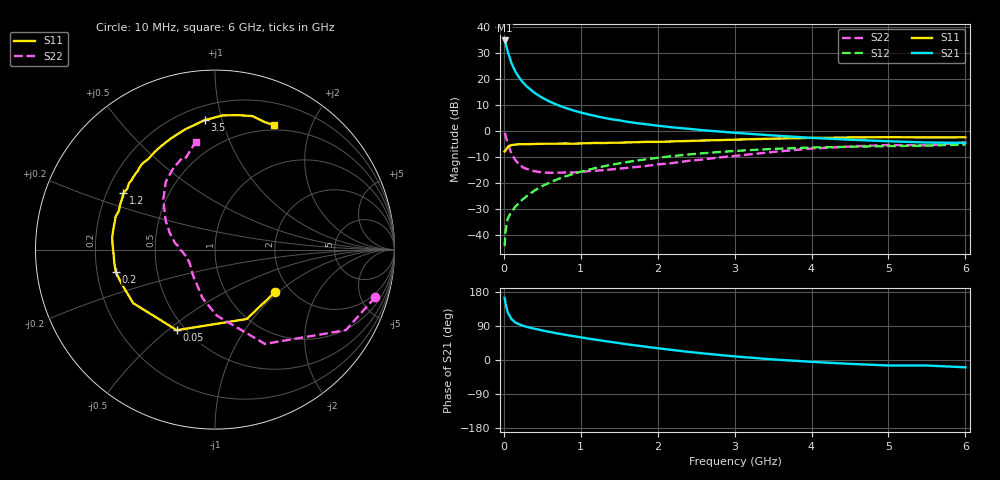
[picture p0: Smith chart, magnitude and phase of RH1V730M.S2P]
! SIEMENS Small Signal Semiconductors
! BFR106
! Si NPN RF Bipolar Junction Transistor in SOT23
! VCE = 1.75 V  IC = 30 mA
! Common Emitter S-Parameters:  August  1996
# GHz  S  MA  R  50
!  f  S11  S21  S12  S22
! GHz  MAG  ANG  MAG  ANG  MAG  ANG  MAG  ANG
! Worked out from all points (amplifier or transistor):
!   36 points, 10 MHz to 6 GHz, reference 50 ohm
!   highest |S21| = 34.9 dB at 10 MHz (marker M1)
!   |S21| within 3 dB of that: start of sweep to 39.23 MHz
!   unconditionally stable (mu >= 1): 282.3 MHz to 2.746 GHz; 5.016 GHz to end of sweep
!   at 250 MHz: K = 0.97, MSG = 22.4 dB, |S12| = -26.1 dB
!   at 1.4 GHz: K = 1.07, MAG = 7.2 dB, |S12| = -12.9 dB
!   at 6 GHz: K = 1.01, MAG = -0.4 dB, |S12| = -5.1 dB
!   S11 on the Smith chart (normalised r, x): 10 MHz: 1.66, -0.95; 50 MHz: 0.45, -0.54; 200 MHz: 0.28, -0.10; 1.2 GHz: 0.27, +0.26; 3.5 GHz: 0.29, +0.88; 6 GHz: 0.44, +1.49
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0.01  0.409 -35.6  55.78 164.0  0.0062 81.6  0.9313 -16.5
0.02  0.4253 -65.4  50.58 151.1  0.0114 69.8  0.8562 -31.6
0.05  0.497 -115.4  34.38 125.6  0.0209 56.2  0.5945 -62.1
0.1  0.5446 -146.8  20.33 107.8  0.0286 54.2  0.3684 -88.3
0.15  0.5546 -160.2  14.05 99.1  0.0357 56.8  0.2794 -104.4
0.2  0.5663 -167.2  10.77 94.0  0.0426 60.0  0.2294 -114.3
0.25  0.566 -172.3  8.629 90.1  0.0498 62.4  0.2019 -124.0
0.3  0.5653 -176.2  7.24 87.3  0.0572 64.5  0.1889 -130.4
0.4  0.5711 177.4  5.489 82.5  0.0729 66.4  0.1708 -141.2
0.5  0.5769 173.2  4.412 78.1  0.0887 67.1  0.1618 -148.5
0.6  0.5775 168.8  3.698 73.9  0.1044 67.0  0.1595 -153.3
0.7  0.5793 165.0  3.201 70.0  0.1202 66.6  0.1607 -157.5
0.9  0.5771 158.2  2.53 63.1  0.1518 64.6  0.1613 -165.4
1.1  0.5905 151.3  2.111 56.4  0.1826 62.2  0.1714 -170.1
1.2  0.5987 148.4  1.956 53.4  0.1976 60.8  0.1752 -172.9
1.6  0.6112 137.0  1.529 41.5  0.2562 54.6  0.1982 178.1
2.2  0.6401 121.7  1.188 26.2  0.3351 44.9  0.2463 164.4
2.8  0.677 107.7  0.992 13.3  0.4 34.9  0.3147 150.3
3.5  0.7232 94.6  0.833 1.5  0.4595 24.0  0.4013 135.9
4.5  0.7604 80.1  0.689 -10.2  0.5054 9.6  0.5103 117.0
5.5  0.7624 68.9  0.609 -14.6  0.5316 0.8  0.5375 107.5
6  0.7668 64.7  0.601 -19.2  0.5577 -6.0  0.6112 100.1
